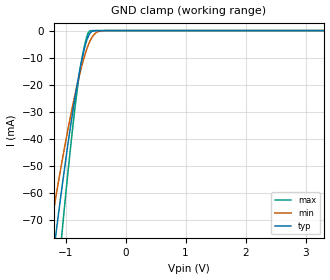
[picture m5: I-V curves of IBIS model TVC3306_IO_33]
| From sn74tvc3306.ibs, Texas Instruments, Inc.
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[Model]   TVC3306_IO_33
Model_type  Terminator
| variable   typ   min   max
C_comp   2.65pF   2.25pF   3.22pF
| C_tri-state   2.65pF   2.25pF   3.22pF
[Temperature Range]   40   100   -40
| Ambient temperature   25   85   -40
[Voltage range]   3.3   3   3.6
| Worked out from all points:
|   GND clamp passes 1 mA (typ) near -0.59 V on its own axis
[GND Clamp]
| TVC3306_IO_33
|   Voltage   I(typ)   I(min)   I(max)
-3.3V     -531.1mA   -415.7mA   -706.1mA
-1.285V   -97.6mA    -78.12mA   -129.7mA
-1.25V    -91.19mA   -73.31mA   -120.9mA
-1.15V    -73.36mA   -59.94mA   -96.23mA
-1.06V    -58.02mA   -48.48mA   -74.88mA
-885mV    -30.71mA   -28.14mA   -36.69mA
-790mV    -17.89mA   -18.51mA   -19.31mA
-680mV    -6.109mA   -9.157mA   -5.225mA
-595mV    -1.038mA   -3.966mA   -104uA
-485mV    -31.54uA   -706.8uA   -862.7nA
-340mV    -334.3nA   -23.07uA   -2.673nA
3.3V      35.08pA    2.903nA    15.72pA
